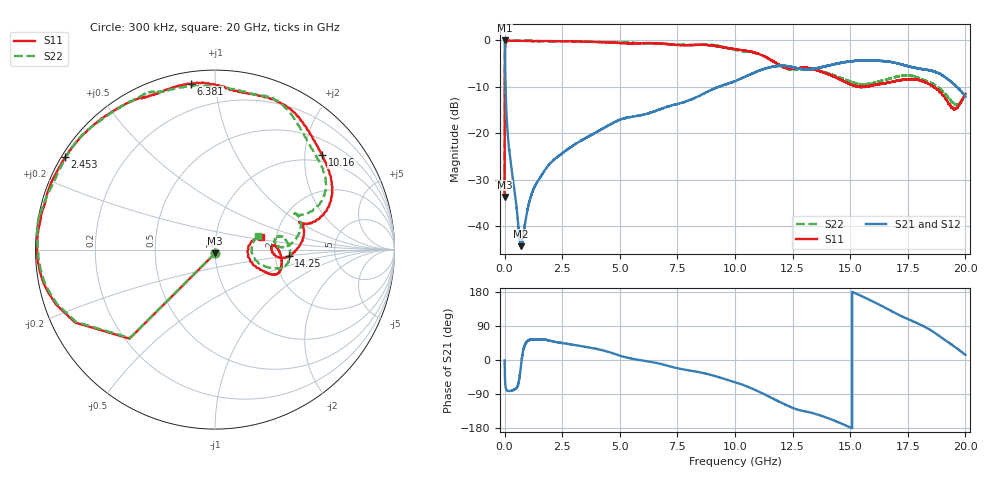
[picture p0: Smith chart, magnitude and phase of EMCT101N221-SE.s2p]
!EMCT101N221
!Johanson Technology Inc.
!www.johansontechnology.com
!Test Board Conditions:
!Substrate Type  RO4350B
!Substrate Thickness  10 mil
!Substrate Dk  3.66
!TL Type: GCPW
!TL Trace Width  22 mil
!TL Gap  14 mil
!PART MODE SINGLE ENDED (AKA BYPASS)
!DUT TOPOLOGY	SERIES-SHUNT
# MHz S  dB  R 50
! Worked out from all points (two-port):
!   20001 points, 300 kHz to 20 GHz, reference 50 ohm
!   highest |S21| = -0.01 dB at 300 kHz (marker M1); lowest = -44.3 dB at 712.3 MHz (marker M2)
!   |S21| within 3 dB of the highest: start of sweep to 13.84 MHz
!   lowest |S11| = -33.7 dB at 300 kHz (marker M3), VSWR 1.04, Z = 50 - j2.06 ohm
!   |S11| at or under -10 dB: 15.41 GHz to 15.56 GHz (147.9 MHz wide, 0.955 % of centre); 15.56 GHz to 15.63 GHz (78.37 MHz wide, 0.503 % of centre); 18.62 GHz to end of sweep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
!   |S22| runs from -33.9 to 0.0 dB; largest |S21 - S12| = 0.015
!   S11 on the Smith chart (normalised r, x): 300 kHz: 1.00, -0.04; 2.453 GHz: 0.01, +0.28; 6.381 GHz: 0.06, +0.86; 10.16 GHz: 0.84, +2.40; 14.25 GHz: 2.38, -0.21; 20 GHz: 1.66, +0.26
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0.3  -33.74 -88.1  -0.01 -1.3  0.01 -1.3  -33.94 -89.6
110.298  -0.12 -174.1  -18.26 -80.7  -18.22 -80.7  -0.19 -174.0
242.296  -0.08 -179.3  -25.44 -81.7  -25.41 -81.8  -0.13 -179.3
712.289  -0.09 173.4  -44.34 -14.7  -44.26 -14.8  -0.04 172.6
1282.281  -0.15 165.4  -31.73 53.8  -31.76 54.2  -0.10 165.3
2453.263  -0.17 148.4  -24.54 45.1  -24.48 44.8  -0.23 150.2
3334.25  -0.26 135.6  -21.55 36.4  -21.57 36.4  -0.19 139.2
5100.224  -0.60 114.9  -16.92 9.7  -16.98 9.9  -0.43 114.1
6381.204  -0.59 98.4  -15.49 -5.4  -15.43 -5.6  -0.69 104.8
6667.2  -0.62 94.4  -14.99 -8.8  -14.96 -9.1  -0.70 100.6
8795.168  -0.99 63.6  -11.09 -36.7  -11.16 -36.8  -0.90 69.7
10000.15  -1.89 43.9  -8.77 -58.6  -8.63 -58.9  -2.02 48.8
10157.15  -1.99 41.3  -8.46 -61.6  -8.34 -62.3  -2.19 45.9
10987.14  -2.83 25.3  -6.65 -82.1  -6.80 -82.2  -2.87 30.7
11732.12  -4.74 15.6  -5.58 -104.5  -5.54 -103.6  -4.70 21.7
13334.1  -6.12 7.4  -6.19 -139.7  -6.20 -139.9  -6.09 14.9
14254.09  -7.70 -5.1  -5.18 -158.6  -5.22 -158.4  -7.44 4.2
15460.07  -10.03 0.3  -4.33 169.6  -4.26 169.4  -9.45 5.9
16667.05  -9.11 0.5  -4.58 133.1  -4.69 133.4  -8.30 10.2
18403.02  -9.38 -24.2  -6.41 81.9  -6.35 81.3  -8.93 -17.1
19478.01  -14.66 -6.5  -9.36 37.4  -9.37 36.7  -13.46 -7.7
20000  -11.52 15.7  -12.16 13.3  -12.29 13.4  -11.88 18.2
